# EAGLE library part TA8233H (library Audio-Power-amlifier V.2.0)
Toshiba 30W BTLx2CH AUDIO POWER AMPLIFIER
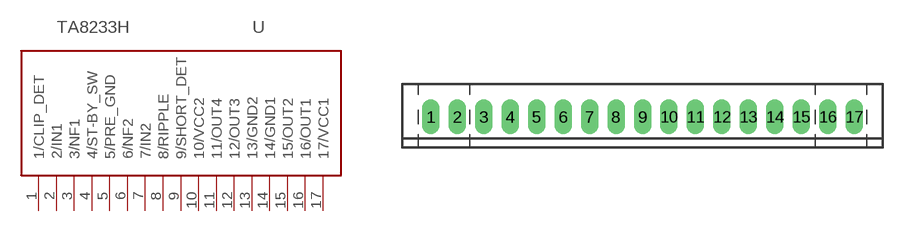
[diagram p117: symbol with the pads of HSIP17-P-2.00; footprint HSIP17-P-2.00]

Designator prefix -

## TA8233H  [HSIP17-P-2.00]
1  1/CLIP_DET
2  2/IN1  in
3  3/NF1  in
4  4/ST-BY_SW
5  5/PRE_GND  pwr
6  6/NF2  in
7  7/IN2  in
8  8/RIPPLE
9  9/SHORT_DET
10  10/VCC2  pwr
11  11/OUT4  out
12  12/OUT3  out
13  13/GND2  pwr
14  14/GND1  pwr
15  15/OUT2  out
16  16/OUT1  out
17  17/VCC1  pwr

## Footprint HSIP17-P-2.00 (pad centres in mm)
HSIP17-P-2.00 Source: http://www.semicon.toshiba.co.jp/td/en/ASSP/Audio_ICs/en_20050517_TA8210ALQ_datasheet.pdf
drill 0.8 pad 1.2 long: 1 -16,0; 2 -14,0; 3 -12,0; 4 -10,0; 5 -8,0; 6 -6,0; 7 -4,0; 8 -2,0; 9 0,0; 10 2,0; 11 4,0; 12 6,0; 13 8,0; 14 10,0; 15 12,0; 16 14,0; 17 16,0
